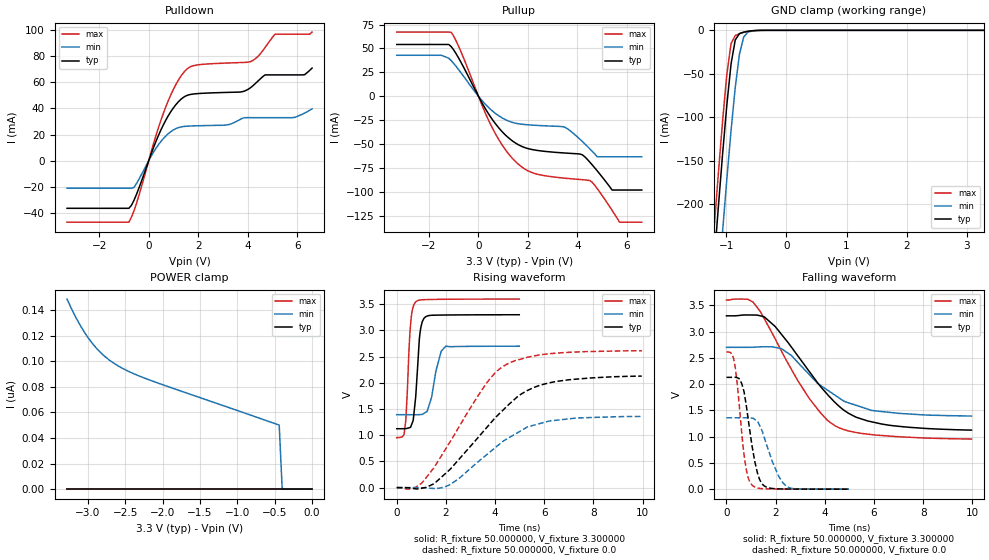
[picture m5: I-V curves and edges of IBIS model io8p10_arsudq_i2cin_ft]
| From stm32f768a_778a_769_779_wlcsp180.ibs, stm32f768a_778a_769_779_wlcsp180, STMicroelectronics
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|   Model io8p10_arsudq_i2cin_ft
[Model]  io8p10_arsudq_i2cin_ft
Model_type I/O
Polarity   Non-Inverting
Enable   Active-Low
Vinl =   0.990000V
Vinh =   2.310000V
Vmeas =  1.650000V
Cref =   40.000000pF
Rref =   100.000000M
Vref =   0.0V
C_comp   2.280000pF   2.217100pF   2.355700pF
[Temperature Range]   25.000000   0.125000k   -40.000000
[Pullup Reference]   3.300000V   2.700000V   3.600000V
[Pulldown Reference]   0.0V   0.0V   0.0V
[POWER Clamp Reference]   3.300000V   2.700000V   3.600000V
[GND Clamp Reference]   0.0V   0.0V   0.0V
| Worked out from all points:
|   slope of the pulldown table from 0 to 0.495 V, typ, clamps not added: 20.9 ohm
|   slope of the pullup table from 0 to 0.495 V, typ, clamps not added: 22.6 ohm
|   GND clamp passes 1 mA (typ) near -0.62 V on its own axis
|   rising waveform, R_fixture 50.000000, V_fixture 3.300000: 20-80 % time 194ps typ, 344ps min, 164ps max; typ from 1.12 V to 3.3 V
|   rising waveform, R_fixture 50.000000, V_fixture 0.0: 20-80 % time 2.52ns typ, 2.29ns min, 2.11ns max; typ from 0 V to 2.13 V
|   falling waveform, R_fixture 50.000000, V_fixture 3.300000: 20-80 % time 2.25ns typ, 2.05ns min, 2.03ns max; typ from 3.3 V to 1.12 V
|   falling waveform, R_fixture 50.000000, V_fixture 0.0: 20-80 % time 433ps typ, 634ps min, 339ps max; typ from 2.13 V to 0 V
[Pulldown]
|Voltage   I(typ)   I(min)   I(max)
-3.3V     -36.46mA   -21.09mA   -47.09mA
-800mV    -36.46mA   -21.09mA   -47.09mA
-600mV    -30.5mA    -20.54mA   -38.69mA
700mV     31.4mA     19.11mA    41.71mA
1.2V      45.15mA    25.37mA    61.75mA
1.6V      50.35mA    26.5mA     71.06mA
3.1V      52.28mA    27.26mA    74.76mA
4.1V      55.7mA     33mA       75.81mA
4.7V      65.72mA    33mA       86.7mA
5.1V      65.72mA    33mA       96.91mA
6.3V      65.88mA    36.51mA    96.91mA
6.6V      70.94mA    39.72mA    98.51mA
[Pullup]
|Voltage   I(typ)   I(min)   I(max)
-3.3V     54.23mA    42.91mA    67.18mA
-1.1V     51.99mA    37.29mA    66.9mA
500mV     -22.07mA   -14mA      -30.03mA
1.5V      -49.1mA    -28.3mA    -68.56mA
2.2V      -56.05mA   -30.32mA   -80.35mA
3.5V      -59.53mA   -32.65mA   -85.92mA
4.2V      -61.43mA   -47.48mA   -87.46mA
4.5V      -69.07mA   -55.12mA   -88.38mA
4.8V      -78.22mA   -63.5mA    -96.83mA
5.4V      -98.3mA    -63.5mA    -119.6mA
5.7V      -98.3mA    -63.5mA    -132mA
6.6V      -98.3mA    -63.5mA    -132mA
[GND_clamp]
|Voltage   I(typ)   I(min)   I(max)
-3.3V     -2.318A    -2.397A    -2.291A
-1.2V     -265.5mA   -356.1mA   -227.2mA
-1.13V    -202.6mA   -292.9mA   -164.1mA
-1.06V    -142.2mA   -231.2mA   -104.1mA
-990mV    -85.98mA   -171.6mA   -50.72mA
-920mV    -38.8mA    -115.5mA   -15.28mA
-850mV    -11.08mA   -65.6mA    -6.001mA
-780mV    -3.782mA   -27.42mA   -3.876mA
-710mV    -2.086mA   -7.69mA    -2.381mA
-640mV    -1.147mA   -2.118mA   -1.22mA
-570mV    -523.9uA   -798.4uA   -476.8uA
3.28V     0A         0A         0A
[POWER_clamp]
|Voltage   I(typ)   I(min)   I(max)
-3.28V    0A         148.5nA    0A
-3.2V     0A         138.6nA    0A
-3.12V    0A         129.7nA    0A
-3.04V    0A         122nA      0A
-2.96V    0A         115.3nA    0A
-2.8V     0A         105.1nA    0A
-2.6V     0A         96.44nA    0A
-2.4V     0A         90.52nA    0A
-2.16V    0A         84.97nA    0A
-440mV    0A         50.04nA    0A
-400mV    0A         0A         0A
0V        0A         0A         0A
[Ramp]
| variable   typ   min   max
dV/dt_r  1.26720/2.50765n   0.81174/2.28853n   1.56390/2.10822n
dV/dt_f  1.28304/2.23594n   0.77796/2.04469n   1.57485/2.02784n
R_load = 50.000000
[Rising Waveform]
R_fixture= 50.000000
V_fixture= 3.300000
V_fixture_min= 2.700000
V_fixture_max= 3.600000
|time   V(typ)   V(min)   V(max)
0s        1.124V     1.392V     954.4mV
300.3ps   1.126V     1.392V     1.022V
370.4ps   1.128V     1.392V     1.295V
540.5ps   1.147V     1.392V     2.987V
760.8ps   1.684V     1.391V     3.538V
940.9ps   2.929V     1.394V     3.581V
1.171ns   3.26V      1.436V     3.588V
1.802ns   3.293V     2.592V     3.594V
2.002ns   3.294V     2.7V       3.595V
4.985ns   3.3V       2.7V       3.599V
[Rising Waveform]
R_fixture= 50.000000
V_fixture= 0.0
V_fixture_min= 0.0
V_fixture_max= 0.0
|time   V(typ)   V(min)   V(max)
0s        344.3uV    197.2uV    670uV
460.5ps   -2.521mV   135uV      -29.38mV
1.021ns   -11.68mV   -1.705mV   87.93mV
1.522ns   76.04mV    -17.08mV   385.3mV
2.142ns   336.1mV    50.68mV    853.5mV
3.644ns   1.138V     622.2mV    1.989V
4.444ns   1.535V     919.5mV    2.347V
5.285ns   1.847V     1.15V      2.484V
6.126ns   1.991V     1.261V     2.551V
9.97ns    2.129V     1.359V     2.612V
[Falling Waveform]
R_fixture= 50.000000
V_fixture= 3.300000
V_fixture_min= 2.700000
V_fixture_max= 3.600000
|time   V(typ)   V(min)   V(max)
0s        3.3V       2.7V       3.599V
880.9ps   3.316V     2.7V       3.612V
1.101ns   3.315V     2.702V     3.551V
1.542ns   3.279V     2.711V     3.242V
2.242ns   2.945V     2.673V     2.625V
3.383ns   2.232V     2.174V     1.718V
4.424ns   1.648V     1.787V     1.206V
5.265ns   1.372V     1.598V     1.079V
6.306ns   1.241V     1.478V     1.022V
9.97ns    1.124V     1.392V     954.4mV
[Falling Waveform]
R_fixture= 50.000000
V_fixture= 0.0
V_fixture_min= 0.0
V_fixture_max= 0.0
|time   V(typ)   V(min)   V(max)
0s        2.129V     1.359V     2.612V
300.3ps   2.13V      1.359V     2.471V
450.5ps   2.119V     1.358V     1.95V
620.6ps   2.012V     1.358V     1.076V
820.8ps   1.55V      1.36V      340.8mV
1.041ns   824.6mV    1.352V     80.07mV
1.451ns   101.6mV    1.111V     10.59mV
1.872ns   12.97mV    518.4mV    4.505mV
2.422ns   2.941mV    64.01mV    2.376mV
4.985ns   344.3uV    197.2uV    670uV
